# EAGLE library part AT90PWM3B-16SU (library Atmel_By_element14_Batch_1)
8-bit Microcontroller with 8K Bytes In-System Programmable Flash
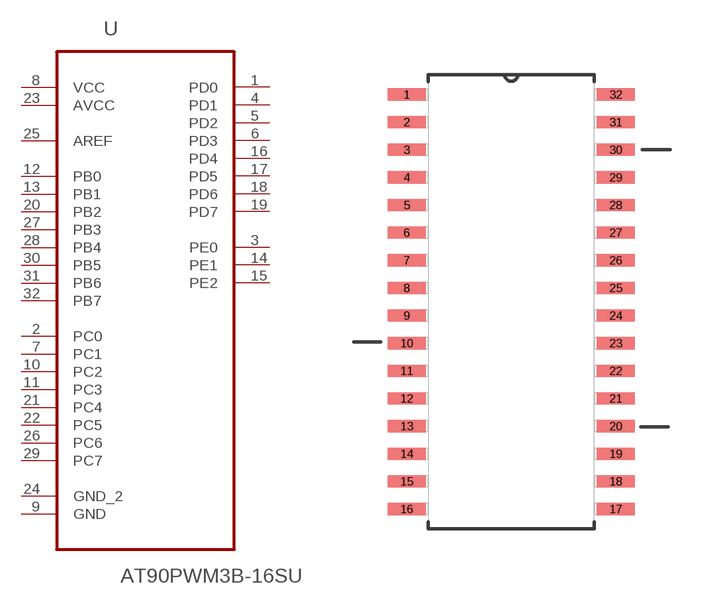
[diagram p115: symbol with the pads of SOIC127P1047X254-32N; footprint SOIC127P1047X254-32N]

Designator prefix U

## AT90PWM3B-16SU (MPN: AT90PWM3B-16SU; OC_FARNELL: 1455069; OC_NEWARK: 58M3864; PACKAGE: SOIC-32; SUPPLIER: Atmel)  [SOIC127P1047X254-32N]
1  PD0
2  PC0
3  PE0
4  PD1
5  PD2
6  PD3
7  PC1
8  VCC  pwr
9  GND  pas
10  PC2
11  PC3
12  PB0
13  PB1
14  PE1
15  PE2
16  PD4
17  PD5
18  PD6
19  PD7
20  PB2
21  PC4
22  PC5
23  AVCC  pwr
24  GND_2  pas
25  AREF  pas
26  PC6
27  PB3
28  PB4
29  PC7
30  PB5
31  PB6
32  PB7

## Footprint SOIC127P1047X254-32N (pad centres in mm)
smd 1.753 x 0.559: 1 -4.801,9.525; 2 -4.801,8.255; 3 -4.801,6.985; 4 -4.801,5.715; 5 -4.801,4.445; 6 -4.801,3.175; 7 -4.801,1.905; 8 -4.801,0.635; 9 -4.801,-0.635; 10 -4.801,-1.905; 11 -4.801,-3.175; 12 -4.801,-4.445; 13 -4.801,-5.715; 14 -4.801,-6.985; 15 -4.801,-8.255; 16 -4.801,-9.525; 17 4.801,-9.525; 18 4.801,-8.255; 19 4.801,-6.985; 20 4.801,-5.715; 21 4.801,-4.445; 22 4.801,-3.175; 23 4.801,-1.905; 24 4.801,-0.635; 25 4.801,0.635; 26 4.801,1.905; 27 4.801,3.175; 28 4.801,4.445; 29 4.801,5.715; 30 4.801,6.985; 31 4.801,8.255; 32 4.801,9.525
